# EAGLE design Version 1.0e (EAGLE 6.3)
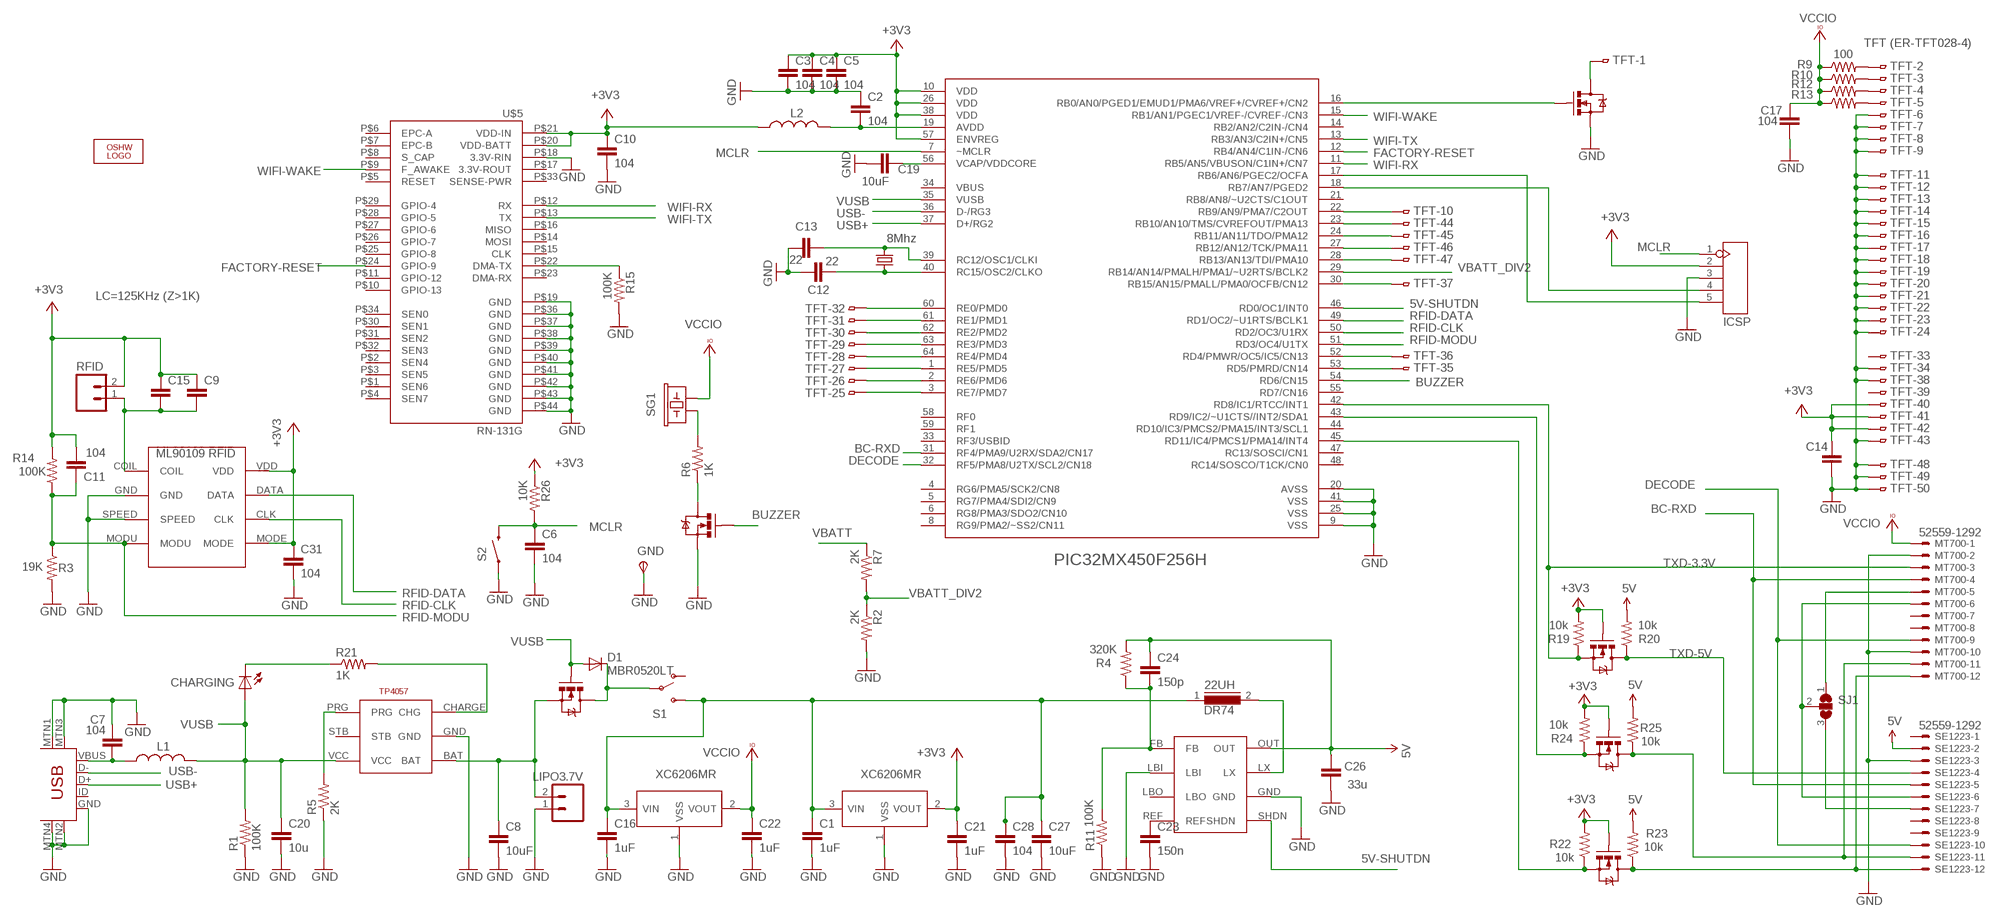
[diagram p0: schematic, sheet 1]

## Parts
22UH  DR74  [DR74]
C1  1uF  C-EUC0805K  [C0805K]
C2  104  CAP0805  [0805]
C3  104  CAP0805  [0805]
C4  104  CAP0805  [0805]
C5  104  CAP0805  [0805]
C6  104  CAP0805  [0805]
C7  104  CAP0805  [0805]
C8  10uF  C-EUC0805K  [C0805K]
C9  LC=125KHz (Z>1K)  CAP0805  [0805]
C10  104  CAP0805  [0805]
C11  104  CAP0805  [0805]
C12  22  CAP0805  [0805]
C13  22  CAP0805  [0805]
C14  104  CAP0805  [0805]
C15  LC=125KHz (Z>1K)  CAP0805  [0805]
C16  1uF  C-EUC0805K  [C0805K]
C17  104  CAP0805  [0805]
C19  10uF  C-EUC0805K  [C0805K]
C20  10u  C-EUC0805K  [C0805K]
C21  1uF  C-EUC0805K  [C0805K]
C22  1uF  C-EUC0805K  [C0805K]
C23  150n  CAP0805  [0805]
C24  150p  CAP0805  [0805]
C26  33u  C-EUC0805K  [C0805K]
C27  10uF  C-EUC0805K  [C0805K]
C28  104  CAP0805  [0805]
C31  104  CAP0805  [0805]
CHARGING  LED1206  [LED-1206]
D1  MBR0520LT  [SOD123]
GND  TPSPAD1-13  [P1-13]
ICSP  HEADER-5P-2.54  [5P-2.54]
L1  INDUCTOR0805  [0805]
L2  INDUCTOR0805  [0805]
LIPO3.7V  M02LOCK  [1X02_LOCK]
LOGO1  LOGO-OSHW-FILLX0200-NT  [OSHW_FILLX200_NOTEXT]
MT700  52559-1292  [52559-1292]
Q1  MOSFET-NCHANNELSMD  [SOT23-3]
Q2  MOSFET-NCHANNELSMD  [SOT23-3]
Q3  MOSFET-NCHANNELSMD  [SOT23-3]
Q7  MOSFET-NCHANNELSMD  [SOT23-3]
Q8  MOSFET-NCHANNELSMD  [SOT23-3]
Q9  MOSFET-NCHANNELSMD  [SOT23-3]
R1  100K  RESISTOR0805-RES  [0805]
R2  2K  RESISTOR0805-RES  [0805]
R3  19K  RESISTOR0805-RES  [0805]
R4  320K  RESISTOR0805-RES  [0805]
R5  2K  RESISTOR0805-RES  [0805]
R6  1K  RESISTOR0805-RES  [0805]
R7  2K  RESISTOR0805-RES  [0805]
R9  100  RESISTOR0805-RES  [0805]
R10  100  RESISTOR0805-RES  [0805]
R11  100K  RESISTOR0805-RES  [0805]
R12  100  RESISTOR0805-RES  [0805]
R13  100  RESISTOR0805-RES  [0805]
R14  100K  RESISTOR0805-RES  [0805]
R15  100K  RESISTOR0805-RES  [0805]
R19  10k  RESISTOR0805-RES  [0805]
R20  10k  RESISTOR0805-RES  [0805]
R21  1K  RESISTOR0805-RES  [0805]
R22  10k  RESISTOR0805-RES  [0805]
R23  10k  RESISTOR0805-RES  [0805]
R24  10k  RESISTOR0805-RES  [0805]
R25  10k  RESISTOR0805-RES  [0805]
R26  10K  RESISTOR0805-RES  [0805]
RFID  M02LOCK  [1X02_LOCK]
S1  SWITCH-SPDT-SMD-A  [SWITCH-SPST-SMD-A]
S2  SWITCH-MOMENTARY-2-SMD-1101NE  [TACTILE-SWITCH-1101NE]
SE1223  52559-1292  [52559-1292]
SG1  BUZZERPTH-NS-KIT  [BUZZER-12MM-NS-KIT]
SJ1  SJ2WW  [SJ_2W]
TFT  TFT (ER-TFT028-4)  FH12-50S-0.5SH  [FH12-50S-0.5SH]
U1  XC6206MR  [SOT23]
U4  XC6206MR  [SOT23]
U$1  MLX90109  [SO-08M]
U$2  USB-MINIB-5PIN  [USB-MINIB]
U$3  NCP1410-MICRO8  [MSOP8]
U$5  RN-131G  [RN-131G]
U$6  TP4057  [SOT23-6]
U$8  PIC32MX450F256H  PIC32MX440F512H  [SQFP-S-10X10-64]
Y1  8Mhz  CRYSTALSMD  [HC49UP]

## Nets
5V: C24.1 C26.1 R4.2 R20.2 R23.2 R25.2 SE1223.2 U$3.OUT
5V-SHUTDN: U$3.SHDN U$8.46(RD0/OC1/INT0)
+3V3: C3.1 C4.1 C5.1 C9.1 C10.1 C11.2 C14.1 C15.1 C21.1 C31.1 ICSP.2 L2.1 Q7.1(G) Q8.1(G) Q9.1(G) R14.2 R19.2 R22.2 R24.2 R26.1 RFID.2 TFT.40 TFT.41 TFT.42 U1.2(VOUT) U$1.MODE U$1.VDD U$5.P$20(VDD-BATT) U$5.P$21(VDD-IN) U$8.10(VDD) U$8.26(VDD) U$8.38(VDD) U$8.57(ENVREG)
BC-RXD: MT700.4 SE1223.5 U$8.31(RF4/PMA9/U2RX/SDA2/CN17)
BUZZER: Q3.1(G) U$8.54(RD6/CN15)
DECODE: MT700.9 SE1223.10 U$8.32(RF5/PMA8/U2TX/SCL2/CN18)
FACTORY-RESET: U$5.P$24(GPIO-9) U$8.12(RB4/AN4/C1IN-/CN6)
GND: C1.2 C2.1 C3.2 C4.2 C5.2 C6.2 C7.2 C8.2 C10.2 C12.1 C13.2 C14.2 C16.2 C17.2 C19.2 C20.2 C21.2 C22.2 C23.2 C26.2 C27.2 C28.2 C31.2 GND.TP(PP) ICSP.3 LIPO3.7V.1 MT700.2 MT700.10 Q1.2(S) Q3.2(S) R1.1 R2.2 R3.2 R5.1 R11.1 R15.2 S2.P$1 SE1223.3 TFT.6 TFT.7 TFT.8 TFT.9 TFT.11 TFT.12 TFT.13 TFT.14 TFT.15 TFT.16 TFT.17 TFT.18 TFT.19 TFT.20 TFT.21 TFT.22 TFT.23 TFT.24 TFT.34 TFT.38 TFT.43 TFT.48 TFT.49 TFT.50 U1.1(VSS) U4.1(VSS) U$1.GND U$1.SPEED U$2.GND U$2.MTN1(MTN2) U$2.MTN2(MTN3) U$2.MTN3(MTN1) U$2.MTN4 U$3.GND U$3.LBI U$5.P$18(3.3V-RIN) U$5.P$19(GND) U$5.P$36(GND) U$5.P$37(GND) U$5.P$38(GND) U$5.P$39(GND) U$5.P$40(GND) U$5.P$41(GND) U$5.P$42(GND) U$5.P$43(GND) U$5.P$44(GND) U$6.GND U$8.9(VSS) U$8.20(AVSS) U$8.25(VSS) U$8.41(VSS)
MCLR: C6.1 ICSP.1 R26.2 S2.P$2 U$8.7(~MCLR)
N$1: C13.1 U$8.39(RC12/OSC1/CLKI) Y1.2
N$2: R15.1 U$5.P$22(DMA-TX)
N$3: C12.2 U$8.40(RC15/OSC2/CLKO) Y1.1
N$4: C7.1 L1.1 U$2.VBUS
N$5: ICSP.4 U$8.18(RB7/AN7/PGED2)
N$6: MT700.6 SE1223.6 SJ1.2
N$7: R5.2 U$6.PRG
N$8: SE1223.7 SJ1.3
N$9: MT700.5 SJ1.1
N$12: 22UH.2 U$3.LX
N$13: C9.2 C15.2 RFID.1 U$1.COIL
N$17: Q8.2(S) R22.1 U$8.45(RD11/IC4/PMCS1/PMA14/INT4)
N$18: C24.2 R4.1 R11.2 U$3.FB
N$19: MT700.12 Q8.3(D) R23.1 SE1223.12
N$20: C23.1 U$3.REF
N$21: R6.2 SG1.-
N$22: R9.2 TFT.2
N$23: R10.2 TFT.3
N$24: R12.2 TFT.4
N$25: R13.2 TFT.5
N$26: Q9.2(S) R24.1 U$8.43(RD9/IC2/~U1CTS//INT2/SDA1)
N$27: MT700.11 Q9.3(D) R25.1 SE1223.11
N$29: TFT.32 U$8.60(RE0/PMD0)
N$30: TFT.31 U$8.61(RE1/PMD1)
N$31: TFT.30 U$8.62(RE2/PMD2)
N$32: TFT.29 U$8.63(RE3/PMD3)
N$33: TFT.28 U$8.64(RE4/PMD4)
N$34: TFT.27 U$8.1(RE5/PMD5)
N$35: TFT.26 U$8.2(RE6/PMD6)
N$36: Q3.3(D) R6.1
N$37: CHARGING.C R21.1
N$38: TFT.25 U$8.3(RE7/PMD7)
N$39: C19.1 U$8.56(VCAP/VDDCORE)
N$40: TFT.44 U$8.23(RB10/AN10/TMS/CVREFOUT/PMA13)
N$41: TFT.45 U$8.24(RB11/AN11/TDO/PMA12)
N$42: TFT.46 U$8.27(RB12/AN12/TCK/PMA11)
N$43: TFT.47 U$8.28(RB13/AN13/TDI/PMA10)
N$45: TFT.37 U$8.30(RB15/AN15/PMALL/PMA0/OCFB/CN12)
N$46: TFT.36 U$8.52(RD4/PMWR/OC5/IC5/CN13)
N$47: TFT.35 U$8.53(RD5/PMRD/CN14)
N$48: TFT.10 U$8.22(RB9/AN9/PMA7/C2OUT)
N$49: D1.C Q2.3(D) S1.2(P)
N$50: R21.2 U$6.CHARGE(CHG)
N$51: C2.2 L2.2 U$8.19(AVDD)
N$52: Q1.1(G) U$8.16(RB0/AN0/PGED1/EMUD1/PMA6/VREF+/CVREF+/CN2)
N$53: Q1.3(D) TFT.1
N$59: ICSP.5 U$8.17(RB6/AN6/PGEC2/OCFA)
RFID-CLK: U$1.CLK U$8.50(RD2/OC3/U1RX)
RFID-DATA: U$1.DATA U$8.49(RD1/OC2/~U1RTS/BCLK1)
RFID-MODU: C11.1 R3.1 R14.1 U$1.MODU U$8.51(RD3/OC4/U1TX)
TXD-3.3V: MT700.3 Q7.2(S) R19.1 U$8.42(RD8/IC1/RTCC/INT1)
TXD-5V: Q7.3(D) R20.1 SE1223.4
USB+: U$2.D+ U$8.37(D+/RG2)
USB-: U$2.D- U$8.36(D-/RG3)
VBAT: 22UH.1 C1.1 C16.1 C27.1 C28.1 S1.3(S) U1.3(VIN) U4.3(VIN)
VBATT: C8.1 LIPO3.7V.2 Q2.2(S) R7.1 U$6.BAT
VBATT_DIV2: R2.1 R7.2 U$8.29(RB14/AN14/PMALH/PMA1/~U2RTS/BCLK2)
VCCIO: C17.1 C22.1 MT700.1 R9.1 R10.1 R12.1 R13.1 SG1.+ U4.2(VOUT)
VUSB: C20.1 CHARGING.A D1.A L1.2 Q2.1(G) R1.2 U$6.VCC U$8.35(VUSB)
WIFI-RX: U$5.P$12(RX) U$8.11(RB5/AN5/VBUSON/C1IN+/CN7)
WIFI-TX: U$5.P$13(TX) U$8.13(RB3/AN3/C2IN+/CN5)
WIFI-WAKE: U$5.P$9(F_AWAKE) U$8.15(RB1/AN1/PGEC1/VREF-/CVREF-/CN3)
Unconnected: MT700.7 MT700.8 S1.1(O) SE1223.1 SE1223.8 SE1223.9 TFT.33 TFT.39 U$2.ID U$3.LBO U$5.P$1(SEN6) U$5.P$2(SEN4) U$5.P$3(SEN5) U$5.P$4(SEN7) U$5.P$5(RESET) U$5.P$6(EPC-A) U$5.P$7(EPC-B) U$5.P$8(S_CAP) U$5.P$10(GPIO-13) U$5.P$11(GPIO-12) U$5.P$14(MOSI) U$5.P$15(CLK) U$5.P$16(MISO) U$5.P$17(3.3V-ROUT) U$5.P$23(DMA-RX) U$5.P$25(GPIO-8) U$5.P$26(GPIO-7) U$5.P$27(GPIO-6) U$5.P$28(GPIO-5) U$5.P$29(GPIO-4) U$5.P$30(SEN1) U$5.P$31(SEN2) U$5.P$32(SEN3) U$5.P$33(SENSE-PWR) U$5.P$34(SEN0) U$6.STB U$8.4(RG6/PMA5/SCK2/CN8) U$8.5(RG7/PMA4/SDI2/CN9) U$8.6(RG8/PMA3/SDO2/CN10) U$8.8(RG9/PMA2/~SS2/CN11) U$8.14(RB2/AN2/C2IN-/CN4) U$8.21(RB8/AN8/~U2CTS/C1OUT) U$8.33(RF3/USBID) U$8.34(VBUS) U$8.44(RD10/IC3/PMCS2/PMA15/INT3/SCL1) U$8.47(RC13/SOSCI/CN1) U$8.48(RC14/SOSCO/T1CK/CN0) U$8.55(RD7/CN16) U$8.58(RF0) U$8.59(RF1)

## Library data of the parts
22UH = inductors:DR74: High Power Density, High Efficiency, Shielded Inductors
C1 C8 C16 C19-C22 C26 C27 = rcl:C-EU: CAPACITOR, European symbol
C2-C7 C9-C15 C17 C23 C24 C28 C31 = SparkFun:CAP: Capacitor
CHARGING = SparkFun:LED: LEDs
D1 = diode:MBR0520LT: SCHOTTKY BARRIER RECTIFIER
GND = testpad:TPS: TEST PIN
ICSP = Connector :HEADER-5P
L1 L2 = SparkFun:INDUCTOR: Inductors
LIPO3.7V RFID = SparkFun:M02: Header 2
LOGO1 = Logo:LOGO-OSHW-FILL; PARTNO: DNP
MT700 SE1223 = con-molex:52559-1292: FFC/FPC-to-Board 0.50mm (.020") SMT, Vertical, ZIF Receptacle Source: http://www.molex.com/product/ffc/52559.html; MPN: 52559-1292; OC_FARNELL: unknown; OC_NEWARK: 91C4526
Q1-Q3 Q7-Q9 = SparkFun:MOSFET-NCHANNEL
R1-R7 R9-R15 R19-R26 = SparkFun:RESISTOR: Resistor
S1 = SparkFun-Electromechanical:SWITCH-SPDT: SPDT Switch Simple slide switch, Spark Fun Electronics SKU : COM-00102 DPDT SMT slide switch, AYZ0202, SWCH-08179
S2 = SparkFun-Electromechanical:SWITCH-MOMENTARY-2: Various NO switches- pushbuttons, reed, etc
SG1 = SparkFun:BUZZER: Buzzer 12mm
SJ1 = jumper:SJ2W: SMD solder JUMPER
TFT = con-hirose:FH12-50S-0.5S: 0.5mm Pitch Connectors For FPC/FFC Source: Data sheet; MPN: FH12-50S-0.5SH(55); OC_FARNELL: 1324557; OC_NEWARK: 34M6181
U1 U4 = IC:XC6206: LOW ESR Cap.Compatible Positive Voltage Regulators
U$1 = boznz:MLX90109: Melexis MLX90109 RFID Reader
U$2 = SparkFun:USB-MINIB: Mini-USB "B" connector with 5th pin broken out. Created new symbol breaking out 5th "ID" pin in mini/micro USB connector spec. See: http://en.wikipedia.org/wiki/Mini_usb#Cables. Uses same footprint as 4-pin symbol. Also added pins to connect to mounting / shield pads if required (probably not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
U$3 = boznz:NCP1410-MICRO8: NCP1410 boost regulator
U$5 = SparkFun:RN-131G: Roving Netowrks WiFLy GSX Module
U$6 = boznz:TP4057
U$8 = SparkFun:PIC32MX440F512H
Y1 = SparkFun:CRYSTAL: Crystals

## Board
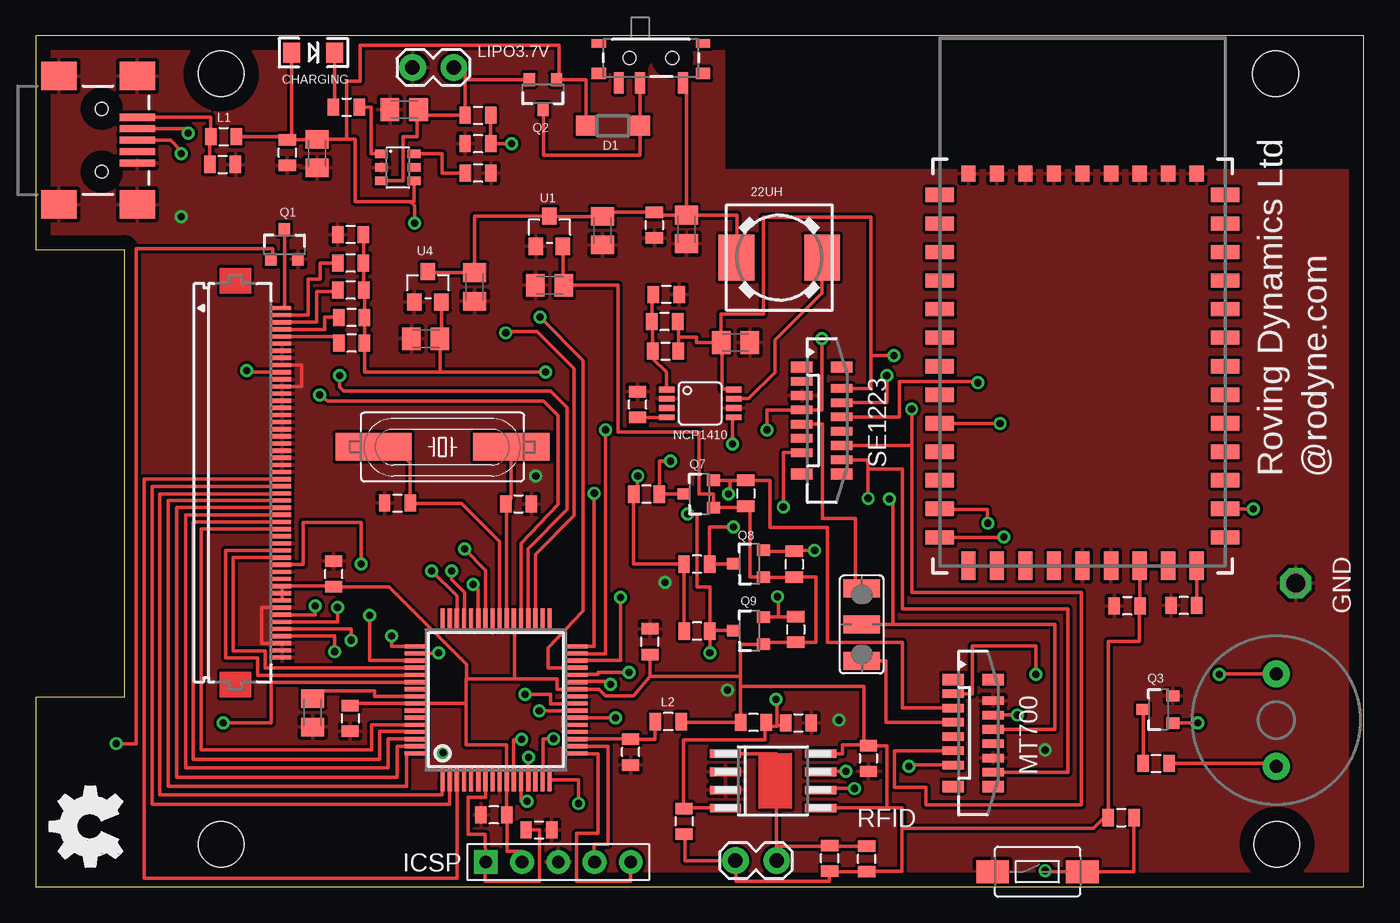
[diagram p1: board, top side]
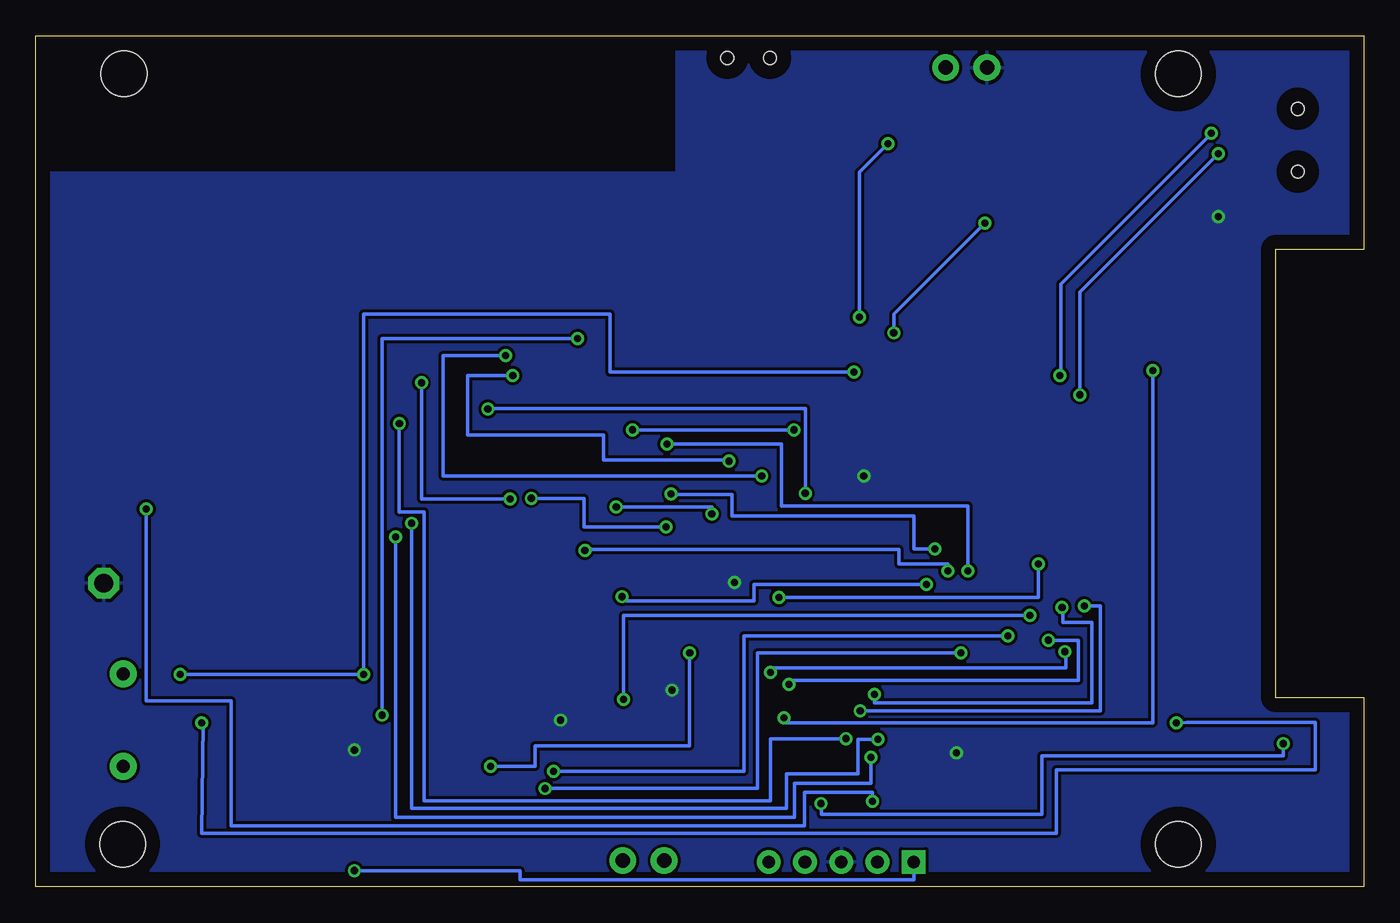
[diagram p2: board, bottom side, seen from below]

Size 93.09 x 59.68 mm. Coordinates in mm from the lower left corner, seen from the top.
Outline: 0,0 93.09,0 93.09,59.68 0,59.68 0,44.69 6.2,44.69 6.2,13.28 0,13.28 0,0
Copper layers (1*16): Top 0.035mm / dielectric 1.5mm / Bottom 0.035mm
Design rules "default": minimum track width 10mil, minimum drill 24mil, track to track 8mil, track to pad 8mil, pad to pad 8mil, via to via 8mil, smd to smd 8mil, copper to edge 40mil, drill to drill 8mil, minimum pad ring 10mil, minimum via ring 8mil, stop-mask expansion 4mil, vias tented up to drill 0mil, thermal gap 10mil
Holes 3.2 mm at 13,3 13,57 86.9,57 87,3

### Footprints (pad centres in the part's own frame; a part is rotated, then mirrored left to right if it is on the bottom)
DR74 = smd 2.5 x 3.25: 1 -3,0; 2 3,0
C0805K = smd 1.3 x 1.6: 1 -1,0; 2 1,0
0805 = smd 0.8 x 1.2: 1 -0.9,0; 2 0.9,0
LED-1206 = smd 1.2 x 1.4: A -1.5,0; C 1.5,0
SOD123 = smd 1.4 x 1.4: A 1.9,0; C -1.9,0
P1-13 = drill 1.321 pad 2.159 octagon: TP 0,0
5P-2.54 = drill 0.889 pad 1.651 square: 1 0,5.08 | drill 0.889 pad 1.651: 2 0,2.54; 3 0,0; 4 0,-2.54; 5 0,-5.08
1X02_LOCK = drill 1.016 pad 1.88: 1 -0.178,0; 2 2.718,0
52559-1292 = smd 0.6 x 1.5: 1 -2.75,-1.4; 2 -2.25,1.4; 3 -1.75,-1.4; 4 -1.25,1.4; 5 -0.75,-1.4; 6 -0.25,1.4; 7 0.25,-1.4; 8 0.75,1.4; 9 1.25,-1.4; 10 1.75,1.4; 11 2.25,-1.4; 12 2.75,1.4 | smd 0.8 x 1.5: M1 -3.75,-1.4; M2 3.75,-1.4; M3 3.75,1.4; M4 -3.75,1.4
SOT23-3 = smd 0.8 x 0.9: 1 -0.95,-1; 2 0.95,-1; 3 0,1.1
SWITCH-SPST-SMD-A = smd 0.7 x 1.5: 1 -2.25,-1.75; 2 -0.75,-1.75; 3 2.25,-1.75 | smd 1 x 0.6: GND1 -3.65,1; GND3 3.65,1 | smd 1 x 0.8: GND2 -3.65,-1.1; GND4 3.65,-1.1 | hole 0.9: -1.5,0; 1.5,0
TACTILE-SWITCH-1101NE = smd 2.3 x 1.6: P$1 -3.15,0; P$2 3.15,0
BUZZER-12MM-NS-KIT = drill 0.9 pad 1.88: + 3.25,0; - -3.25,0
SJ_2W = smd 1.27 x 2.54: 1 -2.54,0; 2 0,0; 3 2.54,0
FH12-50S-0.5SH = smd 0.3 x 1.3: 1 -12.25,3.25; 2 -11.75,3.25; 3 -11.25,3.25; 4 -10.75,3.25; 5 -10.25,3.25; 6 -9.75,3.25; 7 -9.25,3.25; 8 -8.75,3.25; 9 -8.25,3.25; 10 -7.75,3.25; 11 -7.25,3.25; 12 -6.75,3.25; 13 -6.25,3.25; 14 -5.75,3.25; 15 -5.25,3.25; 16 -4.75,3.25; 17 -4.25,3.25; 18 -3.75,3.25; 19 -3.25,3.25; 20 -2.75,3.25; 21 -2.25,3.25; 22 -1.75,3.25; 23 -1.25,3.25; 24 -0.75,3.25; 25 -0.25,3.25; 26 0.25,3.25; 27 0.75,3.25; 28 1.25,3.25; 29 1.75,3.25; 30 2.25,3.25; 31 2.75,3.25; 32 3.25,3.25; 33 3.75,3.25; 34 4.25,3.25; 35 4.75,3.25; 36 5.25,3.25; 37 5.75,3.25; 38 6.25,3.25; 39 6.75,3.25; 40 7.25,3.25; 41 7.75,3.25; 42 8.25,3.25; 43 8.75,3.25; 44 9.25,3.25; 45 9.75,3.25; 46 10.25,3.25; 47 10.75,3.25; 48 11.25,3.25; 49 11.75,3.25; 50 12.25,3.25
SOT23 = smd 1.016 x 1.2: 1 -0.95,-1.06; 2 0.95,-1.06; 3 0,1.06
SO-08M = smd 0.6 x 2.2: CLK 0.635,3.33; COIL -1.905,-3.33; DATA -0.635,3.33; GND -0.635,-3.33; MODE 1.905,3.33; MODU 1.905,-3.33; SPEED 0.635,-3.33; VDD -1.905,3.33
USB-MINIB = smd 2.5 x 0.5: D+ 2.5,0; D- 2.5,0.8; GND 2.5,-1.6; ID 2.5,-0.8; VBUS 2.5,1.6 | smd 2.5 x 2: MTN1 -3,4.5; MTN2 2.5,4.5; MTN3 -3,-4.5; MTN4 2.5,-4.5 | hole 0.9: 0,2.2; 0,-2.2
MSOP8 = smd 1.1 x 0.4: FB -2.477,0.975; GND 2.223,-0.325; LBI -2.477,0.325; LBO -2.477,-0.325; LX 2.223,0.325; OUT 2.223,0.975; REF -2.477,-0.975; SHDN 2.223,-0.975
RN-131G = smd 2 x 1: P$1 -10,11; P$2 -10,9; P$3 -10,7; P$4 -10,5; P$5 -10,3; P$6 -10,1; P$7 -10,-1; P$8 -10,-3; P$9 -10,-5; P$10 -10,-7; P$11 -10,-9; P$12 -10,-11; P$13 -10,-13; P$23 10,-13; P$24 10,-11; P$25 10,-9; P$26 10,-7; P$27 10,-5; P$28 10,-3; P$29 10,-1; P$30 10,1; P$31 10,3; P$32 10,5; P$33 10,7; P$34 10,9; P$35 10,11 | smd 1 x 2: P$14 -8,-15; P$15 -6,-15; P$16 -4,-15; P$17 -2,-15; P$18 0,-15; P$19 2,-15; P$20 4,-15; P$21 6,-15; P$22 8,-15 | smd 1 x 1.11: P$36 8,12.492; P$37 6,12.492; P$38 4,12.492; P$39 2,12.492; P$40 0,12.492; P$41 -2,12.492; P$42 -4,12.492; P$43 -6,12.492; P$44 -8,12.492
SOT23-6 = smd 0.6 x 0.9: BAT 0.95,-1.15; CHARGE -0.95,-1.15; GND 0,-1.15; PRG -0.95,1.15; STB 0,1.15; VCC 0.95,1.15
SQFP-S-10X10-64 = smd 0.3 x 1.6: 1 -3.75,-5.6; 2 -3.25,-5.6; 3 -2.75,-5.6; 4 -2.25,-5.6; 5 -1.75,-5.6; 6 -1.25,-5.6; 7 -0.75,-5.6; 8 -0.25,-5.6; 9 0.25,-5.6; 10 0.75,-5.6; 11 1.25,-5.6; 12 1.75,-5.6; 13 2.25,-5.6; 14 2.75,-5.6; 15 3.25,-5.6; 16 3.75,-5.6; 33 3.75,5.6; 34 3.25,5.6; 35 2.75,5.6; 36 2.25,5.6; 37 1.75,5.6; 38 1.25,5.6; 39 0.75,5.6; 40 0.25,5.6; 41 -0.25,5.6; 42 -0.75,5.6; 43 -1.25,5.6; 44 -1.75,5.6; 45 -2.25,5.6; 46 -2.75,5.6; 47 -3.25,5.6; 48 -3.75,5.6 | smd 1.6 x 0.3: 17 5.6,-3.75; 18 5.6,-3.25; 19 5.6,-2.75; 20 5.6,-2.25; 21 5.6,-1.75; 22 5.6,-1.25; 23 5.6,-0.75; 24 5.6,-0.25; 25 5.6,0.25; 26 5.6,0.75; 27 5.6,1.25; 28 5.6,1.75; 29 5.6,2.25; 30 5.6,2.75; 31 5.6,3.25; 32 5.6,3.75; 49 -5.6,3.75; 50 -5.6,3.25; 51 -5.6,2.75; 52 -5.6,2.25; 53 -5.6,1.75; 54 -5.6,1.25; 55 -5.6,0.75; 56 -5.6,0.25; 57 -5.6,-0.25; 58 -5.6,-0.75; 59 -5.6,-1.25; 60 -5.6,-1.75; 61 -5.6,-2.25; 62 -5.6,-2.75; 63 -5.6,-3.25; 64 -5.6,-3.75
HC49UP = smd 5.334 x 1.93: 1 -4.826,0; 2 4.826,0

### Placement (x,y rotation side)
22UH  52.12,44.12 0 top
C1  30.77,42.07 270 top
C2  41.7,9.46 90 top
C3  43.05,17.2 90 top
C4  32.11,5.05 180 top
C5  22.05,11.82 270 top
C6  35.27,4 0 top
C7  13.11,50.65 0 top
C8  25.84,54.48 180 top
C9  55.65,2.02 90 top
C10  76.5,19.7 180 top
C11  45.45,4.6 270 top
C12  25.36,26.91 0 top
C13  33.85,26.86 0 top
C14  20.89,21.94 90 top
C15  58.25,1.97 90 top
C16  39.72,46.01 270 top
C17  22.07,45.74 180 top
C19  19.42,12.22 270 top
C20  19.72,51.42 270 top
C21  36.03,42.18 180 top
C22  27.34,38.43 180 top
C23  42.19,33.82 90 top
C24  44.09,39.64 180 top
C26  49.05,38.17 0 top
C27  45.62,46.1 270 top
C28  43.36,46.4 270 top
C31  58.36,9.01 270 top
CHARGING  19.45,58.5 0 top
D1  40.46,53.38 180 top
GND  88.32,21.3 0 top
ICSP  36.63,1.75 90 top
L1  13.17,52.6 0 top
L2  44.34,11.59 180 top
LIPO3.7V  26.59,57.45 0 top
LOGO1  6.07,1.41 90 top
MT700  65.7,10.8 270 top
Q1  17.43,45 0 top
Q2  35.56,55.6 180 top
Q3  78.7,12.45 90 top
Q7  46.52,27.55 90 top
Q8  50.02,22.66 90 top
Q9  50.02,17.97 90 top
R1  17.64,51.48 90 top
R2  31,52.1 180 top
R3  53.46,11.51 0 top
R4  44.15,37.56 0 top
R5  31.01,50.04 180 top
R6  78.53,8.66 0 top
R7  31,54.1 0 top
R9  22.08,43.74 180 top
R10  22.09,41.84 180 top
R11  44.2,41.54 180 top
R12  22.14,39.93 180 top
R13  22.15,38.13 180 top
R14  50.31,11.53 180 top
R15  80.47,19.73 180 top
R19  49.77,27.6 270 top
R20  42.81,27.53 180 top
R21  21.78,54.67 0 top
R22  53.17,22.63 270 top
R23  46.34,22.63 180 top
R24  53.27,18.05 270 top
R25  46.36,17.93 180 top
R26  76.08,4.87 0 top
RFID  51.76,1.85 180 top
S1  43.12,58.12 0 top
S2  70.22,1.07 0 top
SE1223  55.1,32.7 270 top
SG1  86.95,11.7 90 top
SJ1  57.9,18.4 90 top
TFT  14.01,28.34 270 top
U1  36.01,45.97 0 top
U4  27.49,42.07 0 top
U$1  51.68,7.44 270 top
U$2  4.63,52.35 0 top
U$3  46.7,33.9 0 top
U$5  73.37,37.51 0 top
U$6  25.38,50.44 270 top
U$8  32.27,13.12 0 top
Y1  28.51,30.85 0 top

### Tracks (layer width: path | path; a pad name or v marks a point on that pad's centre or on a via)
5V  (via drill 0.5)
  Top 0.254: C24.1 45.05,39.64 45.05,38.55 | 45.05,38.55 R4.2 | C26.1 46.3,38.17 46.3,38.55 45.05,38.55 | C26.1 48.1,38.17 48.1,34.9 48.92,34.9 U$3.OUT | R25.2 45.44,17.93 R23.2 41.91,22.63 R20.2 42.2,27.53 v42.2,28.8 | SE1223.2 58.55,34.95 58.55,37.25 | 58.55,37.25 58.55,46.95 51,46.95 51,40.15 48.05,40.15 C26.1 | v60.15,37.25 58.55,37.25
  Bottom 0.254: v42.2,28.8 64.55,28.8 64.55,37.25 v60.15,37.25
5V-SHUTDN  (via drill 0.5)
  Top 0.254: U$3.SHDN 48.85,32.92 v48.85,31.05 | v27.75,22.15 29.52,20.4 U$8.46
  Bottom 0.254: v48.85,31.05 40.8,31.05 40.8,26.7 27.75,26.7 v27.75,22.15
+3V3
  Top 0.254: C5.1 22.05,12.87 U$8.57 30.15,12.87 | 30.15,12.87 30.15,9.95 33.02,9.95 U$8.10 C4.1 33.05,5.25 33.05,2.5 34.04,2.5 ICSP.2 | TFT.42 TFT.41 TFT.40 20.89,21.09 C14.1 24.76,21.04 30.2,15.6 30.2,14.65 30.15,14.6 | U1.2 36.96,42.18 C21.1 40.8,42.18 40.8,31.9 46.5,31.9 46.5,27.55 47.52,27.55 Q7.1 49.77,26.6 R19.2 50.05,26.7 50.05,21.75 51.02,21.75 Q8.1 53.17,21.71 R22.2 54.7,21.73 54.7,17.15 R24.2 51.02,17.15 Q9.1 49.41,17.02 49.41,14.75 | 49.41,14.75 49.41,14.05 | 49.41,14.05 R14.2 45.24,11.53 L2.1 | C3.1 43.05,14.75 | 43.05,14.75 49.41,14.75 | C31.1 58.05,9.91 58.05,14.05 49.41,14.05 | U$1.VDD 56.55,9.35 56.55,9.95 58.06,9.95 C31.1 | U$1.MODE | C11.2 45.5,3.7 45.5,1.85 RFID.2 49.1,1.85 49.1,0.4 55.65,0.4 C9.1 55.65,1.07 C15.1 58.25,1.1 60.7,1.1 60.7,4 | 33.55,14.6 36.55,14.6 36.55,13.87 U$8.26 39.48,13.87 39.95,13.4 41.9,13.4 43.05,14.75 | 33.55,14.6 30.15,14.6 | 30.15,14.6 30.15,12.87 | U$5.P$21 U$5.P$20 77.4,22.51 C10.1 77.35,19.7 77.35,17.2 75.17,17.2 R26.1 74.92,4.87 74.15,4.1 60.8,4.1 60.7,4 | U$8.38 33.55,18.72 33.55,14.6 | 60.7,4 60.7,5.54 U$1.MODE | U$1.MODE 59.65,5.54 59.65,9.9 58.06,9.9 C31.1
BC-RXD  (via drill 0.5)
  Top 0.254: v55.1,38.45 55.1,33.45 SE1223.5 51.25,33.45 v51.25,32.05 | v68.8,12.05 MT700.4 | v39.95,32.05 39.95,16.35 37.87,16.35 U$8.31
  Bottom 0.254: v55.1,38.45 68.8,38.45 v68.8,12.05 | v51.25,32.05 v39.95,32.05
BUZZER  (via drill 0.5)
  Top 0.254: Q3.1 v81.45,11.5 | v13.15,11.5 16.5,11.5 16.5,14.35 26.67,14.35 U$8.54
  Bottom 0.254: v81.45,11.5 81.35,11.5 81.45,3.75 21.55,3.75 21.55,8.2 3.4,8.2 3.4,11.55 12.4,11.55 v13.15,11.5
DECODE  (via drill 0.5)
  Top 0.254: MT700.9 60.2,9.55 60.2,7 62.4,7 62.4,5.75 73.3,5.75 73.3,20.65 61.4,20.65 61.4,30.95 | 61.4,30.95 SE1223.10 | U$8.32 39.15,16.87 v39.15,27.6 | v61.4,33.5 61.4,30.95
  Bottom 0.254: v39.15,27.6 39.15,33.55 61.4,33.55 v61.4,33.5
FACTORY-RESET  (via drill 0.5)
  Top 0.254: U$5.P$24 85,26.51 v85.35,26.5 | v34.45,6 34.02,6 U$8.12
  Bottom 0.254: v85.35,26.5 85.35,13.05 79.4,13.05 79.4,4.3 39.2,4.3 39.2,6.65 34.45,6.65 v34.45,6
GND  (via drill 0.5)
  Top 0.254: TFT.48 15.85,17.09 15.85,19.6 TFT.43 | TFT.9 18.65,36.59 18.65,35.1 TFT.12
  other vias: 28.55,9.4 70.75,9.6 56.3,11.7 35.05,28.8 44.1,21.35 48.5,13.8 10.2,47
  pour Top: 0,59.65 48.2,59.65 48.2,50.2 93.2,50.2 93.2,-0.05 0,-0.05
  pour Bottom: -0.35,59.95 48.15,59.95 48.15,50.05 93.2,50.05 93.4,-0.95 -0.2,-0.95 -0.4,59.55
MCLR  (via drill 0.5)
  Top 0.254: U$8.7 31.55,7.52 31.55,6.3 30.3,6.3 30.3,3.7 31.5,3.7 ICSP.1 31.5,0.4 35.3,0.4 35.3,4 C6.1 | R26.2 76.98,1.07 S2.P$2 70.75,1.07 v70.75,1.15
  Bottom 0.254: v70.75,1.15 59.15,1.15 59.15,0.5 31.55,0.5 ICSP.1
N$1
  Top 0.254: Y1.2 33.34,27.25 C13.1 33.02,26.79 U$8.39
N$2
  Top 0.254: R15.1 U$5.P$22
N$3
  Top 0.254: U$8.40 32.52,24.23 29.85,26.9 C12.2 26.26,29.74 25.2,30.8 23.73,30.8 Y1.1
N$4
  Top 0.254: U$2.VBUS 12.27,53.95 L1.1 12.21,52.6 C7.1
N$5
  Top 0.254: U$8.18 40.1,9.87 40.1,3 39.12,3 ICSP.4
N$6  (via drill 0.5)
  Top 0.254: 60.1,18.4 71.45,18.4 71.45,11.05 MT700.6 | SJ1.2 60.1,18.4 | 60.1,18.4 60.1,27.2 v59.85,27.2 | v66.05,35.35 66.1,35.45 60.55,35.45 60.55,32.95 SE1223.6
  Bottom 0.254: v59.85,27.2 66.05,27.2 v66.05,35.35
N$7
  Top 0.254: R5.2 28.5,50.04 28.5,51.4 U$6.PRG
N$8
  Top 0.254: SJ1.3 57.45,20.94 57.45,25.85 55.15,25.85 55.15,32.45 SE1223.7
N$9
  Top 0.254: SJ1.1 59.6,15.86 59.6,11.55 MT700.5
N$12
  Top 0.254: U$3.LX 49.98,34.23 51.8,36.05 51.8,38.35 55.1,41.65 55.1,44.1 22UH.2
N$13
  Top 0.254: C15.2 55.65,2.87 | 55.65,2.87 C9.2 | 55.65,2.87 51.94,2.87 | 51.94,2.87 51.94,2.65 RFID.1 | U$1.COIL 51.94,9.35 51.94,2.87
N$17  (via drill 0.5)
  Top 0.254: Q8.2 51.02,23.53 R22.1 53.17,23.6 v54.6,23.6 | U$8.45 30.05,18.72 30.05,20.65 29.15,21.55 v29.15,22.15
  Bottom 0.254: v29.15,22.15 29.15,22.65 32.6,22.65 32.6,23.65 54.6,23.65 v54.6,23.6
N$18
  Top 0.254: R11.2 43.19,41.54 C24.2 43.25,39.64 R4.1 43.25,37.05 44.2,36.1 44.2,34.9 U$3.FB
N$19  (via drill 0.5)
  Top 0.254: Q8.3 47.24,22.66 R23.1 47.24,25.25 v48.9,25.25 | SE1223.12 58.35,29.95 58.35,29.3 | 58.35,29.3 v58.35,27.25 | MT700.12 72.35,8.05 72.35,19.5 60.75,19.5 60.75,29.3 58.35,29.3
  Bottom 0.254: v58.35,27.25 54.65,27.25 54.65,25.25 v48.9,25.25
N$20
  Top 0.254: C23.1 U$3.REF
N$21
  Top 0.254: R6.2 86.95,8.66 SG1.-
N$22
  Top 0.254: TFT.2 19.1,40.09 19.1,42.6 19.95,42.6 19.95,43.75 R9.2
N$23
  Top 0.254: TFT.3 19.7,39.59 19.7,41.75 21.19,41.75 R10.2
N$24
  Top 0.254: TFT.4 20.25,39.09 20.25,39.95 21.24,39.95 R12.2
N$25
  Top 0.254: TFT.5 21.25,38.59 R13.2
N$26  (via drill 0.5)
  Top 0.254: R24.1 52.05,18.95 | 52.05,18.95 51.02,18.95 Q9.2 | U$8.43 31,18.72 31,20.85 v30.65,21.2 | v52,20.35 52.05,20.35 52.05,18.95
  Bottom 0.254: v52,20.35 52,20.05 42.75,20.05 42.75,21.2 v30.65,21.2
N$27  (via drill 0.5)
  Top 0.254: Q9.3 47.26,17.97 R25.1 | MT700.11 61.3,8.55 v61.2,8.45 | v47.25,16.4 v47.26,16.4 R25.1 | SE1223.11 52.4,30.45 v52.4,26.65 | R25.1 47.26,21.05 46.35,21.05 46.35,26.15 v45.7,26.15
  Bottom 0.254: v61.2,8.45 58.1,8.45 58.1,9.9 47.25,9.9 v47.25,16.4 | v52.4,26.65 45.7,26.65 v45.7,26.15
N$29
  Top 0.254: TFT.32 11.6,25.1 11.6,9.6 23.55,9.6 23.55,11.37 U$8.60
N$30
  Top 0.254: TFT.31 11.05,25.59 11.05,8.95 24.1,8.95 24.1,10.9 26.67,10.9 U$8.61
N$31
  Top 0.254: TFT.30 10.5,26.09 10.5,8.35 24.7,8.35 24.7,10.4 26.67,10.4 U$8.62
N$32
  Top 0.254: TFT.29 9.9,26.6 9.9,7.7 25.35,7.7 25.35,9.87 U$8.63
N$33
  Top 0.254: TFT.28 9.3,27.09 9.3,7.05 26,7.05 26,9.35 26.67,9.35 U$8.64
N$34
  Top 0.254: U$8.1 28.5,7.52 28.5,6.45 8.7,6.45 8.7,27.55 17.26,27.55 TFT.27
N$35
  Top 0.254: TFT.26 8.15,28.09 8.15,5.8 29.02,5.8 U$8.2
N$36
  Top 0.254: Q3.3 77.63,12.45 R6.1
N$37
  Top 0.254: R21.1 20.95,54.67 CHARGING.C
N$38
  Top 0.254: U$8.3 29.55,7.52 29.55,0.6 7.6,0.6 7.6,28.6 TFT.25
N$39
  Top 0.254: U$8.56 23.75,13.37 23.75,13.75 19.42,13.75 C19.1
N$40  (via drill 0.5)
  Top 0.254: TFT.44 19.6,19.09 v19.6,19.7 | v35.3,12.35 37.87,12.35 U$8.23
  Bottom 0.254: v19.6,19.7 18.45,19.7 18.45,12.35 v35.3,12.35
N$41  (via drill 0.5)
  Top 0.254: TFT.45 21.15,18.59 v21.15,19.6 | v34.3,13.5 36.1,13.5 36.1,12.85 37.87,12.85 U$8.24
  Bottom 0.254: v21.15,19.6 21.1,19.6 21.1,18.55 19.05,18.55 19.05,12.9 34.3,12.9 v34.3,13.5
N$42  (via drill 0.5)
  Top 0.254: TFT.46 22.1,18.09 v22.1,17.3 | v40.3,14.2 40.3,14.4 37.87,14.4 U$8.27
  Bottom 0.254: v22.1,17.3 20,17.3 20,14.5 40.3,14.5 v40.3,14.2
N$43  (via drill 0.5)
  Top 0.254: TFT.47 20.95,17.59 v20.95,16.5 | v41.6,15.05 39.4,15.05 39.4,14.9 37.87,14.9 U$8.28
  Bottom 0.254: v20.95,16.5 20.9,16.5 20.9,15.35 41.45,15.35 v41.6,15.05
N$45  (via drill 0.5)
  Top 0.254: U$8.30 41,15.87 v41,20.3 | v22.8,22.65 22.8,25.55 18.75,25.55 18.75,22.6 TFT.37
  Bottom 0.254: v41,20.3 22.8,20.3 v22.8,22.65
N$46
  Top 0.254: U$8.52 26.67,15.35 16.1,15.35 16.1,16.55 13.85,16.55 13.85,23.09 TFT.36
N$47
  Top 0.254: U$8.53 26.67,14.85 15.55,14.85 15.55,16.05 13.3,16.05 13.3,23.59 TFT.35
N$48  (via drill 0.5)
  Top 0.254: TFT.10 14.8,36.09 v14.8,36.2 | v40.65,11.85 37.87,11.85 U$8.22
  Bottom 0.254: v14.8,36.2 14.8,11.5 40.65,11.5 v40.65,11.85
N$49
  Top 0.254: Q2.3 35.6,54.5 35.6,51.3 42.36,51.3 D1.C S1.2
N$50
  Top 0.254: R21.2 23.5,54.67 23.5,51.4 U$6.CHARGE
N$51
  Top 0.254: L2.2 43.4,11.59 43.4,10.35 C2.2 U$8.19
N$52  (via drill 0.5)
  Top 0.254: Q1.1 16.6,44 16.6,44.75 7.05,44.75 7.05,10.05 v5.65,10.05 | U$8.16 38.05,7.52 v38.05,5.85
  Bottom 0.254: v38.05,5.85 38,5.85 38,5.1 22.55,5.1 22.55,9.2 5.65,9.2 v5.65,10.05
N$53
  Top 0.254: Q1.3 17.45,46.1 17.45,41.1 17.46,40.65 TFT.1
N$59
  Top 0.254: ICSP.5 41.7,1.6 41.7,0.4 37.9,0.4 37.9,3.75 39.4,3.75 39.4,9.35 37.87,9.35 U$8.17
RFID-CLK  (via drill 0.5)
  Top 0.254: U$8.50 28.25,16.37 v28.25,16.4 | v57.4,6.9 55,6.9 55,6.75 U$1.CLK
  Bottom 0.254: v28.25,16.4 42.5,16.4 42.5,6.9 v57.4,6.9
RFID-DATA  (via drill 0.5)
  Top 0.254: U$8.49 24.95,16.87 v24.95,17.6 | v56.8,8.1 55.01,8.1 U$1.DATA
  Bottom 0.254: v24.95,17.6 43.45,17.6 43.45,8.1 v56.8,8.1
RFID-MODU  (via drill 0.5)
  Top 0.254: R3.1 51.95,11.26 | 51.95,11.26 51.26,11.26 R14.1 51.2,11.23 51.13,11.23 51.1,10.3 45.4,10.3 45.4,5.55 C11.1 45.45,5.54 U$1.MODU | U$8.51 23.4,15.87 v23.4,19.05 | v51.9,13.15 51.95,12.75 51.95,11.26
  Bottom 0.254: v23.4,19.05 51.9,19.05 v51.9,13.15
TXD-3.3V  (via drill 0.5)
  Top 0.254: MT700.3 60.75,12.55 60.75,17.15 55.5,17.15 55.5,25.2 51.45,25.2 51.45,28.5 R19.1 48.65,28.5 | 48.65,28.5 Q7.2 | U$8.42 31.55,18.72 31.55,22.2 v30.05,23.7 | v48.55,27.55 48.65,27.55 48.65,28.5
  Bottom 0.254: v48.55,27.55 48.55,27.5 44.3,27.5 44.3,26 31.55,26 31.55,23.7 v30.05,23.7
TXD-5V  (via drill 0.5)
  Top 0.254: Q7.3 43.71,27.55 R20.1 43.71,29.85 v44.5,29.85 | SE1223.4 59.65,33.95 v59.65,35.85
  Bottom 0.254: v59.65,35.85 62.8,35.85 62.8,31.7 53.3,31.7 53.3,29.95 44.5,29.95 v44.5,29.85
USB+  (via drill 0.5)
  Top 0.254: U$8.37 34.02,24.07 36.6,26.8 36.6,33.05 35.6,34.05 20.45,34.05 v19.9,34.5 | v10.2,51.4 10.2,51.6 9.45,52.35 U$2.D+
  Bottom 0.254: v19.9,34.5 19.9,41.7 v10.2,51.4
USB-  (via drill 0.5)
  Top 0.254: U$2.D- 10.4,53.15 v10.7,52.85 | v21.3,35.85 21.3,35.05 21.6,34.75 36.1,34.75 37.25,33.6 37.25,26.45 34.5,23.7 34.5,18.74 U$8.36
  Bottom 0.254: v10.7,52.85 10.7,52.8 21.25,42.25 21.25,35.9 v21.3,35.85
VBAT
  Top 0.254: S1.3 45.62,56.37 C27.1 | 22UH.1 49.15,44.12 49.15,47.1 C27.1 | C27.1 43.36,47.1 C28.1 39.72,47.3 C16.1 36.01,47.01 U1.3 30.77,47.03 C1.1 27.49,43.07 U4.3
VBATT
  Top 0.254: Q2.2 30.1,56.6 | 30.1,56.6 R7.1 26.84,54.1 C8.1 26.75,54.48 26.75,52.6 25.75,52.6 25.75,49.5 U$6.BAT | LIPO3.7V.2 30.1,57.45 30.1,56.6
VBATT_DIV2  (via drill 0.5)
  Top 0.254: R7.2 R2.1 v33.35,52.1 | U$8.29 35.92,15.37 35.9,15.35 35.9,16.75 38.35,19.35 38.35,36.9 v35.35,39.95
  Bottom 0.254: v35.35,39.95 35.35,50.1 v33.35,52.1
VCCIO  (via drill 0.5)
  Top 0.254: C17.1 R9.1 R10.1 23.04,41.84 R12.1 R13.1 23.05,36.1 28.34,36.1 | 28.34,36.1 C22.1 28.44,38.43 U4.2 | SG1.+ 82.95,14.95 v82.95,14.9 | v70.1,14.9 70.1,16.9 65.65,16.9 65.65,13.55 MT700.1 | 28.34,36.1 v35.75,36.1
  Bottom 0.254: v82.95,14.9 v70.1,14.9 70.1,40.15 52.85,40.15 52.85,36.1 v35.75,36.1
VUSB  (via drill 0.5)
  Top 0.254: L1.2 17.64,52.6 R1.2 | R1.2 19.72,52.38 C20.1 21.8,52.42 | R1.2 17.95,52.38 CHARGING.A | 21.8,52.42 22.4,52.42 22.4,48.05 26.25,48.05 | 26.25,48.05 26.53,48.05 U$6.VCC | D1.A 38.56,56.6 Q2.1 36.7,56.6 36.7,59 22.75,59 22.75,56.5 21.8,56.5 21.8,52.42 | U$8.35 35.02,23.32 37.75,26.05 37.75,36.35 35.15,38.95 33.05,38.95 v32.95,38.85 | v26.55,46.55 26.55,47.75 26.25,48.05
  Bottom 0.254: v32.95,38.85 32.95,40.15 v26.55,46.55
WIFI-RX  (via drill 0.5)
  Top 0.254: U$8.11 33.5,7.52 33.5,10.3 34.05,10.3 v34.05,10.35 | v66.75,25.5 66.7,25.5 66.7,26.45 63.37,26.45 U$5.P$12
  Bottom 0.254: v34.05,10.35 35.45,10.35 35.45,7.95 40.45,7.95 40.45,5.5 66.75,5.5 v66.75,25.5
WIFI-TX  (via drill 0.5)
  Top 0.254: U$5.P$13 67.85,24.51 v67.85,24.55 | v34.55,9.1 34.52,9.1 U$8.13
  Bottom 0.254: v67.85,24.55 67.85,4.9 39.9,4.9 39.9,7.25 34.55,7.25 v34.55,9.1
WIFI-WAKE  (via drill 0.5)
  Top 0.254: U$8.15 35.55,7.52 35.55,10.4 v36.3,10.4 | v67.6,32.5 U$5.P$9
  Bottom 0.254: v36.3,10.4 41.6,10.4 41.6,6.05 65.85,6.05 65.85,26.3 67.6,26.3 v67.6,32.5

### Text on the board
tPlace: Roving Dynamics Ltd | @rodyne.com
tValues: + | Install dashed parts / only if option used. | 4 x 100 | SE | MT

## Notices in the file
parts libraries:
SparkFun: Licensing: CC v3.0 Share-Alike You are welcome to use this library for commercial purposes.
